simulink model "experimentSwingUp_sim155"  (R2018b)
settings: Solver=ode4  StartTime=0.0  StopTime=inf  FixedStep=1e-3  RelTol=1e-3
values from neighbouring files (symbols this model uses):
  K = lqr(sysd, Q_lqr, R_lqr)    [mainSkript_provedeniExperimentSwingUp.m]    (also in makeFBL.m = [0; -d_2*g*sin(th_1); -d_3*g*sin(th_2)]; mainSkript_simulaceLQG.m = lqr(sysd, Qk, Rk); mainSkript_LQGexperiment.m = lqr(sysd, Q, R); mainSkript_LQGexperiment_integral.m = lqr(sysd, Q, R))
  K1 = [K1(1 : idxL-rez_1); K1(idxL : idxH); K1(idxH+rez_2 : end)]    [mainSkript_provedeniExperimentSwingUp.m]    (also in mainSkript_provedeniSimulaceSwingUp.m = [K1(1 : idxL-rez); K1(idxL : idxH); K1(idxH+rez : end)])
  K2 = [K2(1 : idxL-rez_1); K2(idxL : idxH); K2(idxH+rez_2 : end)]    [mainSkript_provedeniExperimentSwingUp.m]    (also in mainSkript_provedeniSimulaceSwingUp.m = [K2(1 : idxL-rez); K2(idxL : idxH); K2(idxH+rez : end)])
  K3 = [K3(1 : idxL-rez_1); K3(idxL : idxH); K3(idxH+rez_2 : end)]    [mainSkript_provedeniExperimentSwingUp.m]    (also in mainSkript_provedeniSimulaceSwingUp.m = [K3(1 : idxL-rez); K3(idxL : idxH); K3(idxH+rez : end)])
  K4 = [K4(1 : idxL-rez_1); K4(idxL : idxH); K4(idxH+rez_2 : end)]    [mainSkript_provedeniExperimentSwingUp.m]    (also in mainSkript_provedeniSimulaceSwingUp.m = [K4(1 : idxL-rez); K4(idxL : idxH); K4(idxH+rez : end)])
  K5 = [K5(1 : idxL-rez_1); K5(idxL : idxH); K5(idxH+rez_2 : end)]    [mainSkript_provedeniExperimentSwingUp.m]    (also in mainSkript_provedeniSimulaceSwingUp.m = [K5(1 : idxL-rez); K5(idxL : idxH); K5(idxH+rez : end)])
  K6 = [K6(1 : idxL-rez_1); K6(idxL : idxH); K6(idxH+rez_2 : end)]    [mainSkript_provedeniExperimentSwingUp.m]    (also in mainSkript_provedeniSimulaceSwingUp.m = [K6(1 : idxL-rez); K6(idxL : idxH); K6(idxH+rez : end)])
  Ki = [Ki(1 : idxL-rez_1); Ki(idxL : idxH); Ki(idxH+rez_2 : end)]    [mainSkript_provedeniExperimentSwingUp.m]    (also in mainSkript_provedeniSimulaceSwingUp.m = [Ki(1 : idxL-rez); Ki(idxL : idxH); Ki(idxH+rez : end)])
  t_FB = [t_FB(1 : idxL-rez_1); t_FB(idxL : idxH); t_FB(idxH+rez_2 : end)]    [mainSkript_provedeniExperimentSwingUp.m]    (also in mainSkript_provedeniSimulaceSwingUp.m = [t_FB(1 : idxL-rez); t_FB(idxL : idxH); t_FB(idxH+rez : end))
  Ts = 1e-3    (= 0.001)    [mainSkript_provedeniExperimentSwingUp.m]    (also in mainSkript_rovniceSystemu.m; mainSkript_simulaceLQG.m; mainSkript_LQGexperiment.m; mainSkript_LQGexperiment_integral.m)
undefined symbols (not defined in the file or in its folder): DiscIntNeverNeededParam, Humusoft, MF624
libraries: sldrtlib x8, simulink x7, powerlib_meascontrol x3, sharedTrackingLibrary x2

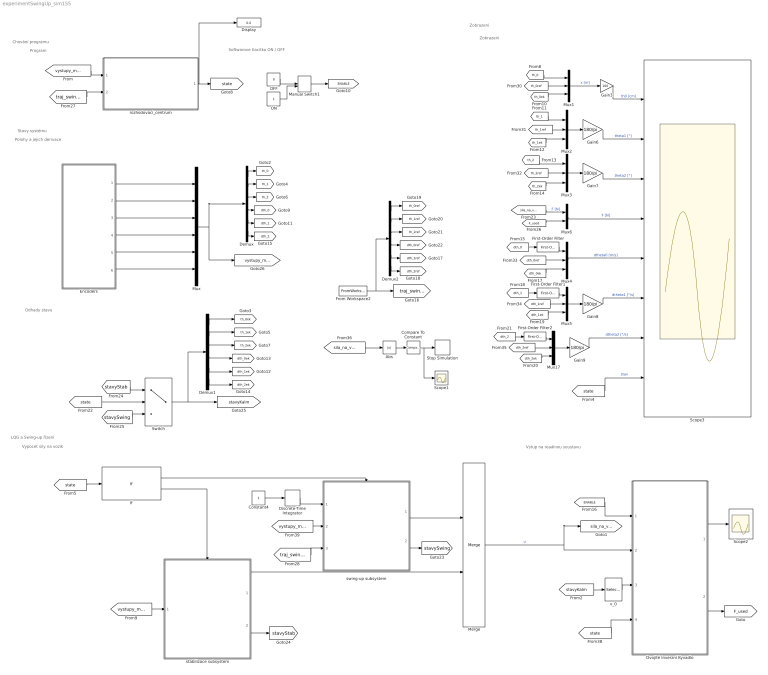
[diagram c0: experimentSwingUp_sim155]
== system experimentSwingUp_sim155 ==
  note: Odhady stavu
  note: Zobrazeni
  note: Chování programu
  note: LQG a Swing-up řízení
  note: Stavy systému
  note: Polohy a jejich derivace
  note: Softwarove tlacitko ON / OFF
  note: Program
  note: Vstup na reaálnou soustavu
  note: Vypocet sily na vozik
  note: Zobrazeni
  Abs : Abs
  Compare To Constant : simulink/Logic and Bit Operations/Compare To Constant  relop=>  const=35  OutDataTypeStr=boolean
  Constant4 : Constant
  Demux : Demux  Outputs=6
  Demux1 : Demux  Outputs=6
  Demux2 : Demux  Outputs=6
  Discrete-Time Integrator : DiscreteIntegrator  SampleTime=Ts  ICPrevOutput=DiscIntNeverNeededParam  ICPrevScaledInput=DiscIntNeverNeededParam
  Display : Display
  Dvojité Inverzní Kyvadlo : Subsystem
  Encoders : Subsystem
  First-Order Filter : powerlib_meascontrol/Filters/First-Order Filter  FilterType=Lowpass  Tc=4e-3  Ts=Ts  Initialize=on  Vac_Init=[0, 0, 60]  Vdc_Init=0  PlotResponse=off  FreqRange="[0,  200,  1]"
  First-Order Filter1 : powerlib_meascontrol/Filters/First-Order Filter  FilterType=Lowpass  Tc=6e-3  Ts=Ts  Initialize=on  Vac_Init=[0, 0, 60]  Vdc_Init=0  PlotResponse=off  FreqRange="[0,  200,  1]"
  First-Order Filter2 : powerlib_meascontrol/Filters/First-Order Filter  FilterType=Lowpass  Tc=6e-3  Ts=Ts  Initialize=on  Vac_Init=[0, 0, 60]  Vdc_Init=0  PlotResponse=off  FreqRange="[0,  200,  1]"
  From Workspace2 : FromWorkspace  VariableName=ref_traj  SampleTime=Ts
  Gain3 : Gain  Gain=100
  Gain{6..9} (4 alike) : Gain  Gain=180/pi
  If : If  IfExpression=u1 == 0  ElseIfExpressions=u1 == 1  ShowElse=off
  Manual Switch1 : ManualSwitch  CurrentSetting=0
  Merge : Merge
  Mux : Mux  Inputs=6
  Mux{1..5,17} (6 alike) : Mux  Inputs=3
  Mux6 : Mux  Inputs=2
  OFF : Constant  Value=0
  ON : Constant
  Scope1 : Scope
  Scope2 : Scope
  Scope3 : Scope  NumInputPorts=8
  Stop Simulation : Stop
  Switch : Switch  Criteria=u2 > Threshold
  rozhodovaci_centrum : Subsystem
  stabilizace subsystem : Subsystem  TreatAsAtomicUnit=on
  swing-up subsystem : Subsystem  TreatAsAtomicUnit=on
  v_0 : Selector  InputPortWidth=6  IndexOptions=Index vector (dialog)  Indices=[4]  OutputSizes=1
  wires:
  OFF/1 -> Manual Switch1/1
  ON/1 -> Manual Switch1/2
  Manual Switch1/1 -> [ENABLE]
  [ENABLE] -> Dvojité Inverzní Kyvadlo/1(ENABLE)
  Dvojité Inverzní Kyvadlo/1(sat_flag) -> Scope2/1
  Dvojité Inverzní Kyvadlo/2(F_used [N]) -> [F_used]
  If/2 -> stabilizace subsystem/Action
  Discrete-Time Integrator/1 -> swing-up subsystem/1(cas Swing-upu [s])
  If/1 -> swing-up subsystem/Action
  stabilizace subsystem/1(sila na vozik [N]) -> Merge/2
  [stavyKalm] -> v_0/1
  [vystupy_mereni] -> rozhodovaci_centrum/1(stavySystemu)
  [state] -> Scope3/8  "stav"
  Mux/1 -> [vystupy_mereni], Demux/1
  Switch/1 -> Demux1/1, [stavyKalm]
  Demux/1 -> [th_0]
  Demux1/1 -> [th_0ek]
  Demux/2 -> [th_1]
  Demux1/2 -> [th_1ek]
  Demux/3 -> [th_2]
  Demux1/3 -> [th_2ek]
  Demux/4 -> [dth_0]
  Demux/5 -> [dth_1]
  Demux1/5 -> [dth_1ek]
  Demux1/4 -> [dth_0ek]
  Demux1/6 -> [dth_2ek]
  Demux/6 -> [dth_2]
  Constant4/1 -> Discrete-Time Integrator/1
  Compare To Constant/1 -> Scope1/1, Stop Simulation/1
  Encoders/1(th0 [m]) -> Mux/1
  Encoders/2(th1 [rad]) -> Mux/2
  Encoders/3(th2 [rad]) -> Mux/3
  Encoders/5(dth1 [rad/s]) -> Mux/5
  Encoders/6(dth2 [rad/s]) -> Mux/6
  Mux17/1 -> Gain9/1
  Gain8/1 -> Scope3/6  "dtheta1 [°/s]"
  [th_2] -> Mux3/1
  [dth_0] -> First-Order Filter/1
  [dth_0ref] -> Mux4/2
  [th_0ref] -> Mux1/2
  [dth_1ref] -> Mux5/2
  Gain7/1 -> Scope3/3  "theta2 [°]"
  Gain6/1 -> Scope3/2  "theta1 [°]"
  Mux5/1 -> Gain8/1
  [th_2ek] -> Mux3/3
  Mux4/1 -> Scope3/5  "dtheta0 [m/s]"
  [th_0] -> Mux1/1
  [th_2ref] -> Mux3/2
  Gain9/1 -> Scope3/7  "dtheta2 [°/s]"
  Mux1/1 -> Gain3/1  "x [m]"
  [dth_2ek] -> Mux17/3
  [dth_1ek] -> Mux5/3
  Mux2/1 -> Gain6/1
  [dth_0ek] -> Mux4/3
  [dth_2ref] -> Mux17/2
  [th_1ref] -> Mux2/2
  [th_1ek] -> Mux2/3
  Mux3/1 -> Gain7/1
  [th_1] -> Mux2/1
  [th_0ek] -> Mux1/3
  Gain3/1 -> Scope3/1  "th0 [cm]"
  [sila_na_vozik] -> Mux6/1  "F [N]"
  Mux6/1 -> Scope3/4  "F [N]"
  [F_used] -> Mux6/2
  [traj_swingUp] -> rozhodovaci_centrum/2(trajektorieSwingUp)
  [traj_swingUp] -> swing-up subsystem/3(trajektorie swing-up)
  Demux2/6 -> [dth_2ref]
  Demux2/5 -> [dth_1ref]
  Demux2/4 -> [dth_0ref]
  Demux2/3 -> [th_2ref]
  Demux2/2 -> [th_1ref]
  Demux2/1 -> [th_0ref]
  From Workspace2/1 -> Demux2/1, [traj_swingUp]
  [state] -> If/1
  Abs/1 -> Compare To Constant/1
  [sila_na_vozik] -> Abs/1
  swing-up subsystem/1(sila na vozik [N]) -> Merge/1
  rozhodovaci_centrum/1(error_state) -> [state], Display/1
  Encoders/4(dth0 [m/s]) -> Mux/4
  First-Order Filter/1 -> Mux4/1
  [dth_1] -> First-Order Filter1/1
  First-Order Filter1/1 -> Mux5/1
  [dth_2] -> First-Order Filter2/1
  First-Order Filter2/1 -> Mux17/1
  [state] -> Dvojité Inverzní Kyvadlo/4(stav)
  [vystupy_mereni] -> swing-up subsystem/2(mereni)
  swing-up subsystem/2(stavyKalm) -> [stavySwing]
  [vystupy_mereni] -> stabilizace subsystem/1(mereni)
  stabilizace subsystem/2(stavy) -> [stavyStab]
  [stavyStab] -> Switch/1
  [state] -> Switch/2
  [stavySwing] -> Switch/3
  v_0/1 -> Dvojité Inverzní Kyvadlo/3(v [m/s])
  Merge/1 -> [sila_na_vozik], Dvojité Inverzní Kyvadlo/2(F_in [N])  "u"

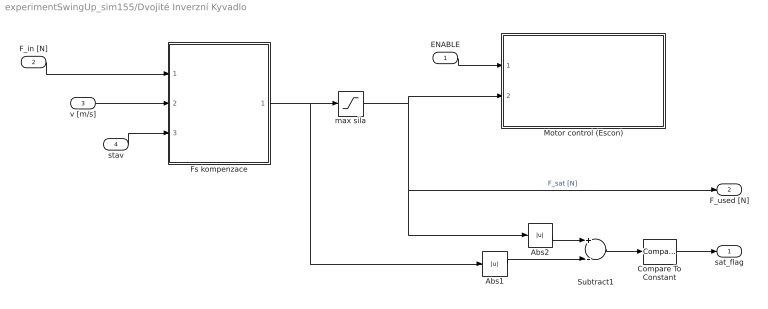
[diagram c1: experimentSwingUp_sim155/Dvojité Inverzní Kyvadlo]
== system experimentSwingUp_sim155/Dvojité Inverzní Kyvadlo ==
  ENABLE : Inport
  F_in [N] : Inport  Port=2
  v [m/s] : Inport  Port=3
  stav : Inport  Port=4
  Abs1 : Abs
  Abs2 : Abs
  Compare To Constant : simulink/Logic and Bit Operations/Compare To Constant  relop=>  const=1e-8  OutDataTypeStr=boolean
  Fs kompenzace : Subsystem
  Motor control (Escon) : Subsystem
  Subtract1 : Sum  Inputs=+-
  max sila : Saturate  UpperLimit=50  LowerLimit=-50
  sat_flag : Outport
  F_used [N] : Outport  Port=2
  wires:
  ENABLE/1 -> Motor control (Escon)/1(ENABLE)
  v [m/s]/1 -> Fs kompenzace/2(v [m/s])
  F_in [N]/1 -> Fs kompenzace/1(F_in [N])
  Compare To Constant/1 -> sat_flag/1
  Subtract1/1 -> Compare To Constant/1
  Abs1/1 -> Subtract1/2
  max sila/1 -> Motor control (Escon)/2(Ref strength [N]), F_used [N]/1, Abs2/1  "F_sat [N]"
  Abs2/1 -> Subtract1/1
  Fs kompenzace/1(F_out [N]) -> Abs1/1, max sila/1
  stav/1 -> Fs kompenzace/3(stav)

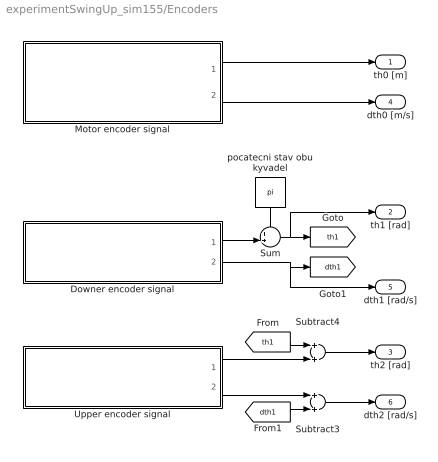
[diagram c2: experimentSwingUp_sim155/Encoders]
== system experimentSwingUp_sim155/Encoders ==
  Downer encoder signal : Subsystem
  Motor encoder signal : Subsystem
  Subtract3 : Sum
  Subtract4 : Sum
  Sum : Sum  Inputs=++|
  Upper encoder signal : Subsystem
  pocatecni stav obu kyvadel : Constant  Value=pi
  th0 [m] : Outport
  th1 [rad] : Outport  Port=2
  th2 [rad] : Outport  Port=3
  dth0 [m/s] : Outport  Port=4
  dth1 [rad/s] : Outport  Port=5
  dth2 [rad/s] : Outport  Port=6
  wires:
  pocatecni stav obu kyvadel/1 -> Sum/1
  Downer encoder signal/1(phi [rad]) -> Sum/2
  Sum/1 -> th1 [rad]/1, [th1]
  Downer encoder signal/2(omega [rad/s]) -> dth1 [rad/s]/1, [dth1]
  Upper encoder signal/1(phi [rad]) -> Subtract4/2
  Upper encoder signal/2(omega [rad/s]) -> Subtract3/1
  [th1] -> Subtract4/1
  [dth1] -> Subtract3/2
  Subtract4/1 -> th2 [rad]/1
  Subtract3/1 -> dth2 [rad/s]/1
  Motor encoder signal/1(x [m]) -> th0 [m]/1
  Motor encoder signal/2(v [m/s]) -> dth0 [m/s]/1

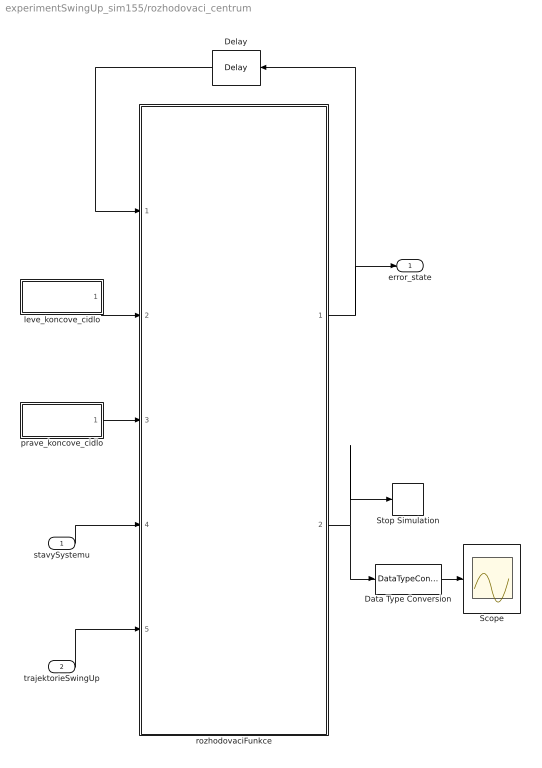
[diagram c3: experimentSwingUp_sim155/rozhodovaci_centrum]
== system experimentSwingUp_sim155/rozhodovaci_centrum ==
  stavySystemu : Inport
  trajektorieSwingUp : Inport  Port=2
  Data Type Conversion : DataTypeConversion  OutDataTypeStr=double
  Delay : Delay  DelayLength=1  InitialCondition=0  UseCircularBuffer=on  SampleTime=Ts
  Scope : Scope
  Stop Simulation : Stop
  leve_koncove_cidlo : Subsystem
  prave_koncove_cidlo : Subsystem
  rozhodovaciFunkce : MATLAB Function  TreatAsAtomicUnit=on
  error_state : Outport
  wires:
  rozhodovaciFunkce/1(state) -> Delay/1, error_state/1
  rozhodovaciFunkce/2(error) -> Stop Simulation/1, Data Type Conversion/1
  Delay/1 -> rozhodovaciFunkce/1(last_state)
  Data Type Conversion/1 -> Scope/1
  leve_koncove_cidlo/1(NOK) -> rozhodovaciFunkce/2(leftSens)
  prave_koncove_cidlo/1(NOK) -> rozhodovaciFunkce/3(rightSens)
  stavySystemu/1 -> rozhodovaciFunkce/4(stavySystemu)
  trajektorieSwingUp/1 -> rozhodovaciFunkce/5(traj)

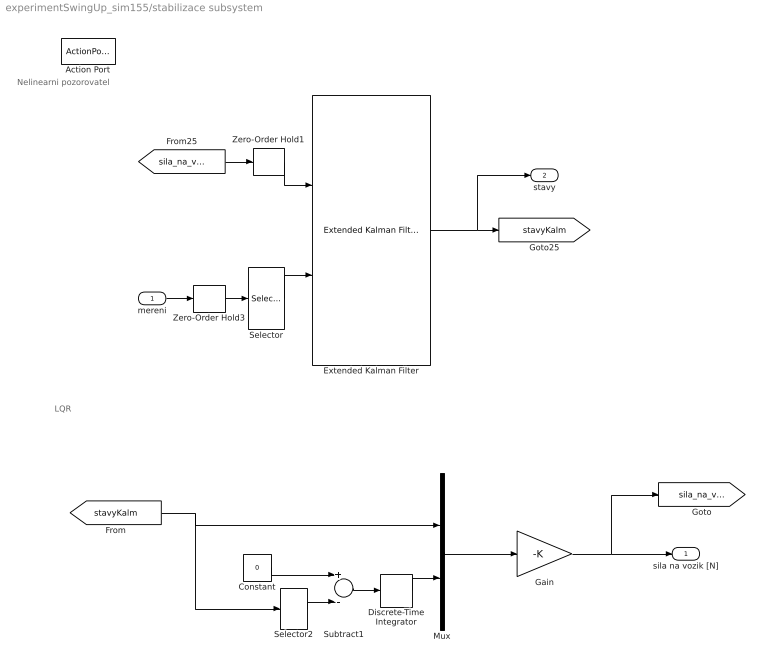
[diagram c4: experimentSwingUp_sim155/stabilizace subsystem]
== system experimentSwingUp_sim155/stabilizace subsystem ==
  note: LQR
  note: Nelinearni pozorovatel
  mereni : Inport
  Action Port : ActionPort  ActionType=elseif
  Constant : Constant  Value=0
  Discrete-Time Integrator : DiscreteIntegrator  SampleTime=Ts  ICPrevOutput=DiscIntNeverNeededParam  ICPrevScaledInput=DiscIntNeverNeededParam
  Extended Kalman Filter : sharedTrackingLibrary/Extended Kalman Filter  StateTransitionFcn=nonLinKalmFcn_pn0  HasStateTransitionJacobianFcn=on  StateTransitionJacobianFcn=countJacobDIP_pn0  HasAdditiveProcessNoise=Additive  ProcessNoise=Q_stab  HasTimeVaryingProcessNoise=off  HasStateTransitionFcnExtraArgument=1  InitialState=q_0  InitialStateCovariance=1e-6*eye(6)  MeasurementFcn1=mereniStavuKalm  HasMeasurementJacobianFcn1=off  HasMeasurementEnablePort1=off  HasAdditiveMeasurementNoise1=Additive  MeasurementNoise1=R_stab  HasTimeVaryingMeasurementNoise1=off  HasMeasurementFcnExtraArgument1=0  MeasurementFcn2=myMeasurementFcn  HasMeasurementJacobianFcn2=off  HasMeasurementEnablePort2=off  HasAdditiveMeasurementNoise2=Additive  MeasurementNoise2=1  HasTimeVaryingMeasurementNoise2=off  HasMeasurementFcnExtraArgument2=0  MeasurementFcn3=myMeasurementFcn  HasMeasurementJacobianFcn3=off  HasMeasurementEnablePort3=off  HasAdditiveMeasurementNoise3=Additive  MeasurementNoise3=1  HasTimeVaryingMeasurementNoise3=off  HasMeasurementFcnExtraArgument3=0  MeasurementFcn4=myMeasurementFcn  HasMeasurementJacobianFcn4=off  HasMeasurementEnablePort4=off  HasAdditiveMeasurementNoise4=Additive  MeasurementNoise4=1  HasTimeVaryingMeasurementNoise4=off  HasMeasurementFcnExtraArgument4=0  MeasurementFcn5=myMeasurementFcn  HasMeasurementJacobianFcn5=off  HasMeasurementEnablePort5=off  HasAdditiveMeasurementNoise5=Additive  MeasurementNoise5=1  HasTimeVaryingMeasurementNoise5=off  HasMeasurementFcnExtraArgument5=0  EnableMultirate=off  StateTransitionFcnSampleTime=1  MeasurementFcn1SampleTime=1  MeasurementFcn2SampleTime=1  MeasurementFcn3SampleTime=1  MeasurementFcn4SampleTime=1  MeasurementFcn5SampleTime=1  UseCurrentEstimator=on  OutputStateCovariance=off  DataType=double  SampleTime=Ts  NumberOfMeasurements=1
  Gain : Gain  Gain=-K  Multiplication=Matrix(K*u) (u vector)
  Mux : Mux  Inputs=2
  Selector : Selector  InputPortWidth=6  IndexOptions=Index vector (dialog)  Indices=[1:3]  OutputSizes=1
  Selector2 : Selector  InputPortWidth=6  IndexOptions=Index vector (dialog)  Indices=[1]  OutputSizes=1
  Subtract1 : Sum  Inputs=+-
  Zero-Order Hold1 : ZeroOrderHold  SampleTime=Ts
  Zero-Order Hold3 : ZeroOrderHold  SampleTime=Ts
  sila na vozik [N] : Outport
  stavy : Outport  Port=2
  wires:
  Selector2/1 -> Subtract1/2
  Subtract1/1 -> Discrete-Time Integrator/1
  Mux/1 -> Gain/1
  Discrete-Time Integrator/1 -> Mux/2
  Constant/1 -> Subtract1/1
  Gain/1 -> [sila_na_vozik], sila na vozik [N]/1
  Zero-Order Hold3/1 -> Selector/1
  [sila_na_vozik] -> Zero-Order Hold1/1
  Selector/1 -> Extended Kalman Filter/2
  mereni/1 -> Zero-Order Hold3/1
  Extended Kalman Filter/1 -> stavy/1, [stavyKalm]
  Zero-Order Hold1/1 -> Extended Kalman Filter/1
  [stavyKalm] -> Selector2/1, Mux/1

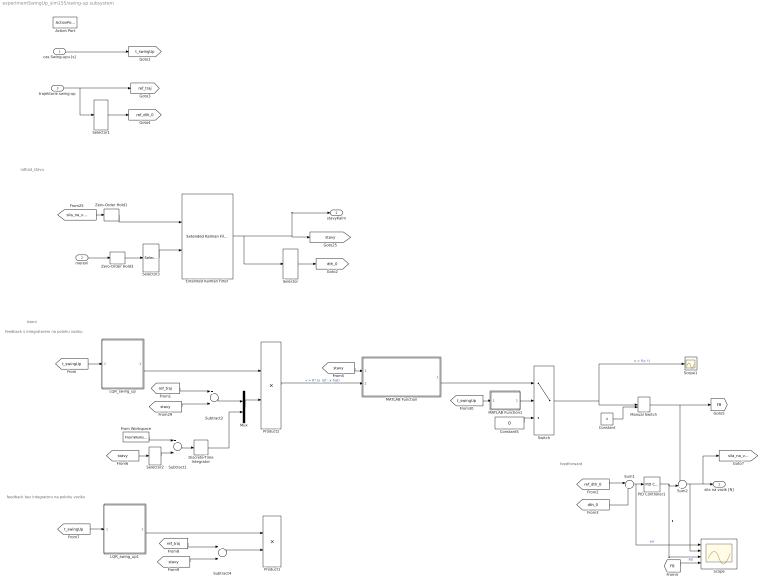
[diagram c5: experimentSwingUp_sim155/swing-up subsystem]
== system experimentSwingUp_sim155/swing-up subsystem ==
  note: odhad_stavu
  note: rizeni
  note: feedback s integratorem na polohu voziku
  note: feedforward
  note: feedback bez integratoru na polohu voziku
  cas Swing-upu [s] : Inport
  mereni : Inport  Port=2
  trajektorie swing-up : Inport  Port=3
  Action Port : ActionPort  ActionType=then
  Constant : Constant  Value=0
  Constant5 : Constant  Value=0
  Discrete-Time Integrator : DiscreteIntegrator  SampleTime=Ts  ICPrevOutput=DiscIntNeverNeededParam  ICPrevScaledInput=DiscIntNeverNeededParam
  Extended Kalman Filter : sharedTrackingLibrary/Extended Kalman Filter  StateTransitionFcn=nonLinKalmFcn_pn155  HasStateTransitionJacobianFcn=on  StateTransitionJacobianFcn=countJacobDIP_pn155  HasAdditiveProcessNoise=Additive  ProcessNoise=Q_swing  HasTimeVaryingProcessNoise=off  HasStateTransitionFcnExtraArgument=1  InitialState=q_0  InitialStateCovariance=1e-6*eye(6)  MeasurementFcn1=mereniStavuKalm  HasMeasurementJacobianFcn1=off  HasMeasurementEnablePort1=off  HasAdditiveMeasurementNoise1=Additive  MeasurementNoise1=R_swing  HasTimeVaryingMeasurementNoise1=off  HasMeasurementFcnExtraArgument1=0  MeasurementFcn2=myMeasurementFcn  HasMeasurementJacobianFcn2=off  HasMeasurementEnablePort2=off  HasAdditiveMeasurementNoise2=Additive  MeasurementNoise2=1  HasTimeVaryingMeasurementNoise2=off  HasMeasurementFcnExtraArgument2=0  MeasurementFcn3=myMeasurementFcn  HasMeasurementJacobianFcn3=off  HasMeasurementEnablePort3=off  HasAdditiveMeasurementNoise3=Additive  MeasurementNoise3=1  HasTimeVaryingMeasurementNoise3=off  HasMeasurementFcnExtraArgument3=0  MeasurementFcn4=myMeasurementFcn  HasMeasurementJacobianFcn4=off  HasMeasurementEnablePort4=off  HasAdditiveMeasurementNoise4=Additive  MeasurementNoise4=1  HasTimeVaryingMeasurementNoise4=off  HasMeasurementFcnExtraArgument4=0  MeasurementFcn5=myMeasurementFcn  HasMeasurementJacobianFcn5=off  HasMeasurementEnablePort5=off  HasAdditiveMeasurementNoise5=Additive  MeasurementNoise5=1  HasTimeVaryingMeasurementNoise5=off  HasMeasurementFcnExtraArgument5=0  EnableMultirate=off  StateTransitionFcnSampleTime=1  MeasurementFcn1SampleTime=1  MeasurementFcn2SampleTime=1  MeasurementFcn3SampleTime=1  MeasurementFcn4SampleTime=1  MeasurementFcn5SampleTime=1  UseCurrentEstimator=on  OutputStateCovariance=off  DataType=double  SampleTime=Ts  NumberOfMeasurements=1
  From Workspace : FromWorkspace  VariableName=theta0_str  SampleTime=Ts
  LQR_swing_up : Subsystem
  LQR_swing_up1 : Subsystem  Commented=on
  MATLAB Function : MATLAB Function  TreatAsAtomicUnit=on
  MATLAB Function1 : MATLAB Function  TreatAsAtomicUnit=on
  Manual Switch : ManualSwitch
  Mux : Mux  Inputs=2
  PID Controller1 : simulink/Continuous/PID Controller  Controller=PID  Form=Parallel  TimeDomain=Discrete-time  SampleTime=Ts  IntegratorMethod=Forward Euler  FilterMethod=Forward Euler  ControllerParametersSource=internal  P=520  I=1610  D=0  UseFilter=on  N=100  TunerSelectOption=Transfer Function Based (PID Tuner App)  InitialConditionSource=internal  InitialConditionForIntegrator=0  InitialConditionForFilter=0  DifferentiatorICPrevScaledInput=0  ExternalReset=none  TrackingMode=off  Kt=1  LimitOutput=off  UpperSaturationLimit=inf  LowerSaturationLimit=-inf  LinearizeAsGain=on  AntiWindupMode=none  Kb=1  POutMin=[]  POutMax=[]  IOutMin=[]  IOutMax=[]  DOutMin=[]  DOutMax=[]  NOutMin=[]  NOutMax=[]  SumOutMin=[]  SumOutMax=[]  SaturationOutMin=[]  SaturationOutMax=[]  PParamMin=[]  PParamMax=[]  IParamMin=[]  IParamMax=[]  DParamMin=[]  DParamMax=[]  NParamMin=[]  NParamMax=[]  KbParamMin=[]  KbParamMax=[]  KtParamMin=[]  KtParamMax=[]  KbOutMin=[]  KbOutMax=[]  KtOutMin=[]  KtOutMax=[]  IntegratorOutMin=[]  IntegratorOutMax=[]  FilterOutMin=[]  FilterOutMax=[]  SumI1OutMin=[]  SumI1OutMax=[]  SumI2OutMin=[]  SumI2OutMax=[]  SumI3OutMin=[]  SumI3OutMax=[]  SumI4OutMin=[]  SumI4OutMax=[]  SumDOutMin=[]  SumDOutMax=[]  DifferentiatorOutMin=[]  DifferentiatorOutMax=[]  FilterDiffOutCoefMin=[]  FilterDiffOutCoefMax=[]  ReciprocalOutMin=[]  ReciprocalOutMax=[]  SumDenOutMin=[]  SumDenOutMax=[]  SumNumOutMin=[]  SumNumOutMax=[]  DivideOutMin=[]  DivideOutMax=[]  IntegratorContinuousStateAttributes=''  IntegratorStateMustResolveToSignalObject=off  IntegratorRTWStateStorageClass=Auto  FilterContinuousStateAttributes=''  FilterStateMustResolveToSignalObject=off  FilterRTWStateStorageClass=Auto  ParallelPVariant=InternalParameters  IdealPVariant=Disabled  IVariant=InternalParameters  DVariant=InternalParameters  IntegratorVariant=Discrete  SatVariant=Disabled  AWVariant=Passthrough  PCopyVariant=Disabled  TRVariant=Disabled  FdbkBlocksVariant=Forward  IdealPFdbkVariant=Disabled  SatFdbkVariant=Disabled  DerivativeFilterVariant=ForwardEulerFilter  NVariant=InternalParameters  NCopyVariant=Disabled  FilterICVariant=InternalICsFilter  IntegratorICVariant=InternalICs  ExternalResetVariant=Disabled  TRSumVariant=Passthrough  SumFdbkVariant=Disabled  SumVariant=Sum_PID
  Product1 : Product  Commented=on  Multiplication=Matrix(*)
  Product2 : Product  Multiplication=Matrix(*)
  Scope : Scope  NumInputPorts=4
  Scope1 : Scope
  Selector : Selector  InputPortWidth=6  IndexOptions=Index vector (dialog)  Indices=[4]  OutputSizes=1
  Selector1 : Selector  InputPortWidth=6  IndexOptions=Index vector (dialog)  Indices=[4]  OutputSizes=1
  Selector2 : Selector  InputPortWidth=6  IndexOptions=Index vector (dialog)  Indices=[1]  OutputSizes=1
  Selector3 : Selector  InputPortWidth=6  IndexOptions=Index vector (dialog)  Indices=[1:3]  OutputSizes=1
  Subtract1 : Sum  Inputs=+-
  Subtract2 : Sum  Inputs=+-
  Subtract4 : Sum  Commented=on  Inputs=+-
  Sum1 : Sum  Inputs=|+-
  Sum2 : Sum  Inputs=++|
  Switch : Switch  Criteria=u2 ~= 0
  Zero-Order Hold1 : ZeroOrderHold  SampleTime=Ts
  Zero-Order Hold3 : ZeroOrderHold  SampleTime=Ts
  sila na vozik [N] : Outport
  stavyKalm : Outport  Port=2
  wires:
  Sum2/1 -> Scope/2, [sila_na_vozik], sila na vozik [N]/1
  Sum1/1 -> Scope/1, PID Controller1/1  "err"
  [ref_dth_0] -> Sum1/1
  PID Controller1/1 -> Scope/3, Sum2/2  "FF"
  [stavy] -> Subtract2/2
  Constant5/1 -> Switch/3
  [t_swingUp] -> MATLAB Function1/1(time)
  [dth_0] -> Sum1/2
  cas Swing-upu [s]/1 -> [t_swingUp]
  [t_swingUp] -> LQR_swing_up/1(t)
  Selector/1 -> [dth_0]
  trajektorie swing-up/1 -> Selector1/1, [ref_traj]
  Selector1/1 -> [ref_dth_0]
  [ref_traj] -> Subtract2/1
  LQR_swing_up/1(K(t)) -> Product2/1
  MATLAB Function1/1(on) -> Switch/2
  Switch/1 -> Scope1/1, Manual Switch/1  "u = f(x, t)"
  Constant/1 -> Manual Switch/2
  Manual Switch/1 -> [FB], Sum2/1
  [FB] -> Scope/4  "FB"
  MATLAB Function/1(u) -> Switch/1
  [stavy] -> MATLAB Function/1(y)
  Mux/1 -> Product2/2
  Subtract2/1 -> Mux/1
  From Workspace/1 -> Subtract1/1
  Selector2/1 -> Subtract1/2
  [stavy] -> Selector2/1
  Subtract1/1 -> Discrete-Time Integrator/1
  Discrete-Time Integrator/1 -> Mux/2
  mereni/1 -> Zero-Order Hold3/1
  Zero-Order Hold3/1 -> Selector3/1
  Selector3/1 -> Extended Kalman Filter/2
  Extended Kalman Filter/1 -> Selector/1, stavyKalm/1, [stavy]
  Zero-Order Hold1/1 -> Extended Kalman Filter/1
  [sila_na_vozik] -> Zero-Order Hold1/1
  [stavy] -> Subtract4/2
  LQR_swing_up1/1(K(t)) -> Product1/1
  [t_swingUp] -> LQR_swing_up1/1(t)
  [ref_traj] -> Subtract4/1
  Subtract4/1 -> Product1/2
  Product2/1 -> MATLAB Function/2(v)  "v = K* (x_ref - x_hat)"

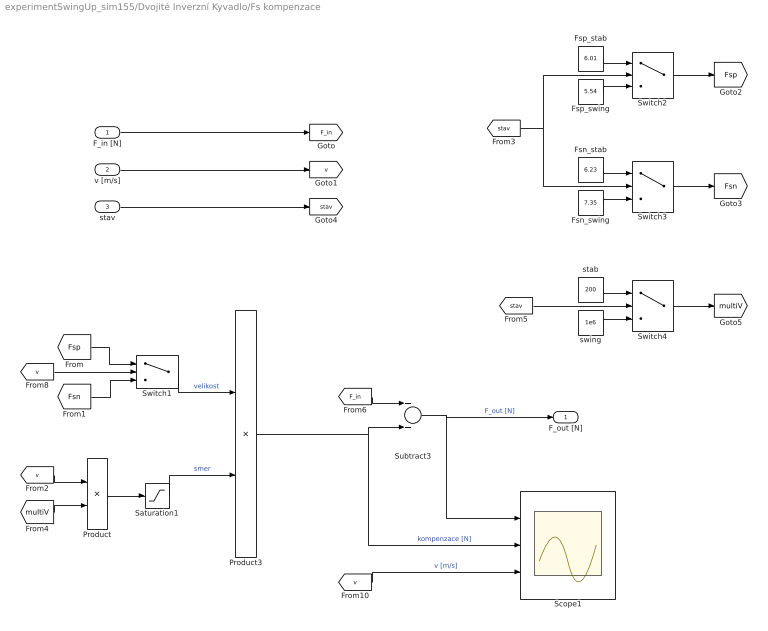
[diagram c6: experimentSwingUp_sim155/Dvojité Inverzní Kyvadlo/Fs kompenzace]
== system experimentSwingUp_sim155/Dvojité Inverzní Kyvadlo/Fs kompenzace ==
  F_in [N] : Inport
  v [m/s] : Inport  Port=2
  stav : Inport  Port=3
  Fsn_stab : Constant  Value=6.23
  Fsn_swing : Constant  Value=7.35
  Fsp_stab : Constant  Value=6.01
  Fsp_swing : Constant  Value=5.54
  Product : Product
  Product3 : Product
  Saturation1 : Saturate  UpperLimit=1  LowerLimit=-1
  Scope1 : Scope  NumInputPorts=3
  Subtract3 : Sum
  Switch1 : Switch
  Switch2 : Switch  Criteria=u2 > Threshold
  Switch3 : Switch  Criteria=u2 > Threshold
  Switch4 : Switch  Criteria=u2 > Threshold
  stab : Constant  Value=200
  swing : Constant  Value=1e6
  F_out [N] : Outport
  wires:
  F_in [N]/1 -> [F_in]
  v [m/s]/1 -> [v]
  [Fsn] -> Switch1/3
  [v] -> Switch1/2
  [Fsp] -> Switch1/1
  [F_in] -> Subtract3/1
  [v] -> Scope1/3  "v [m/s]"
  Subtract3/1 -> F_out [N]/1, Scope1/1  "F_out [N]"
  Saturation1/1 -> Product3/2  "smer"
  Product3/1 -> Subtract3/2, Scope1/2  "kompenzace [N]"
  Product/1 -> Saturation1/1
  Switch1/1 -> Product3/1  "velikost"
  [stav] -> Switch3/2, Switch2/2
  Fsp_swing/1 -> Switch2/3
  Fsn_swing/1 -> Switch3/3
  Switch2/1 -> [Fsp]
  Switch3/1 -> [Fsn]
  Fsp_stab/1 -> Switch2/1
  Fsn_stab/1 -> Switch3/1
  stav/1 -> [stav]
  [v] -> Product/1
  [multiV] -> Product/2
  [stav] -> Switch4/2
  swing/1 -> Switch4/3
  stab/1 -> Switch4/1
  Switch4/1 -> [multiV]

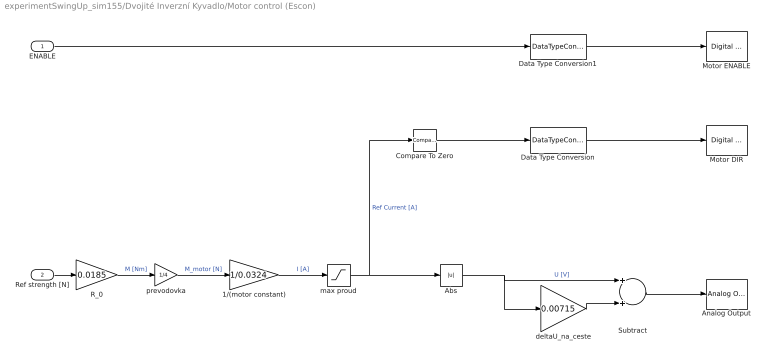
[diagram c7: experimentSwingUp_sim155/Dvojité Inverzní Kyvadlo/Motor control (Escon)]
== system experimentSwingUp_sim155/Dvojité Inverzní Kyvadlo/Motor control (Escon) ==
  ENABLE : Inport
  Ref strength [N] : Inport  Port=2
  1/(motor constant) : Gain  Gain=1/0.0324
  Abs : Abs
  Analog Output : sldrtlib/Analog Output  SampleTime=Ts  MaxMissedTicks=1e6  ShowMissedTicks=off  YieldWhenWaiting=off  DrvName=Humusoft/MF624  DrvAddress=4294967295  DrvOptions=0  Channels=6  RangeMode=1  VoltRange=1  InitialValue=0  FinalValue=0
  Compare To Zero : simulink/Logic and Bit Operations/Compare To Zero  relop=>=  OutDataTypeStr=boolean
  Data Type Conversion : DataTypeConversion  OutDataTypeStr=boolean
  Data Type Conversion1 : DataTypeConversion  OutDataTypeStr=boolean
  Motor DIR : sldrtlib/Digital Output  SampleTime=Ts  MaxMissedTicks=1e6  ShowMissedTicks=off  YieldWhenWaiting=off  DrvName=Humusoft/MF624  DrvAddress=4294967295  DrvOptions=0  Channels=5  BitMode=1  InitialValue=0  FinalValue=0
  Motor ENABLE : sldrtlib/Digital Output  SampleTime=Ts  MaxMissedTicks=1e6  ShowMissedTicks=off  YieldWhenWaiting=off  DrvName=Humusoft/MF624  DrvAddress=4294967295  DrvOptions=0  Channels=2  BitMode=1  InitialValue=0  FinalValue=0
  R_0 : Gain  Gain=0.0185
  Subtract : Sum
  deltaU_na_ceste : Gain  Gain=0.00715
  max proud : Saturate  UpperLimit=10  LowerLimit=-10
  prevodovka : Gain  Gain=1/4
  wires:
  Compare To Zero/1 -> Data Type Conversion/1
  Data Type Conversion1/1 -> Motor ENABLE/1
  1/(motor constant)/1 -> max proud/1  "I [A]"
  max proud/1 -> Abs/1, Compare To Zero/1  "Ref Current [A]"
  Ref strength [N]/1 -> R_0/1
  ENABLE/1 -> Data Type Conversion1/1
  R_0/1 -> prevodovka/1  "M [Nm]"
  prevodovka/1 -> 1/(motor constant)/1  "M_motor [N]"
  Data Type Conversion/1 -> Motor DIR/1
  Subtract/1 -> Analog Output/1
  deltaU_na_ceste/1 -> Subtract/2
  Abs/1 -> Subtract/1, deltaU_na_ceste/1  "U [V]"

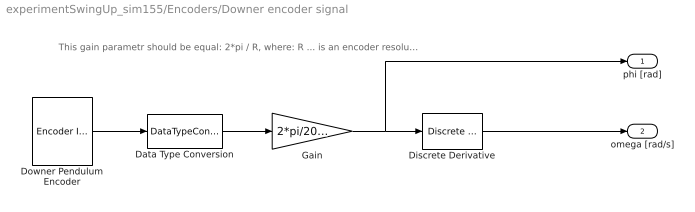
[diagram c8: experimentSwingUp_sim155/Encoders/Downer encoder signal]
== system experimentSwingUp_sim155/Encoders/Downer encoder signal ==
  note: This gain parametr should be equal: 2*pi / R, where: R ... is an encoder resolution
  Data Type Conversion : DataTypeConversion  OutDataTypeStr=double
  Discrete Derivative : simulink/Discrete/Discrete Derivative  gainval=1.0  ICPrevScaledInput=0.0  OutMin=[]  OutMax=[]  OutDataType=fixdt(1, 16)  OutScaling=2^-10  DoSatur=off
  Downer Pendulum Encoder : sldrtlib/Encoder Input  SampleTime=Ts  MaxMissedTicks=1e8  ShowMissedTicks=off  YieldWhenWaiting=off  DrvName=Humusoft/MF624  DrvAddress=4294967295  DrvOptions=0  Channels=2  QuadMode=3  IndexPulse=1  InputFilter=Inf  DataType=7
  Gain : Gain  Gain=2*pi/2048
  phi [rad] : Outport
  omega [rad/s] : Outport  Port=2
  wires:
  Downer Pendulum Encoder/1 -> Data Type Conversion/1
  Discrete Derivative/1 -> omega [rad/s]/1
  Data Type Conversion/1 -> Gain/1
  Gain/1 -> Discrete Derivative/1, phi [rad]/1

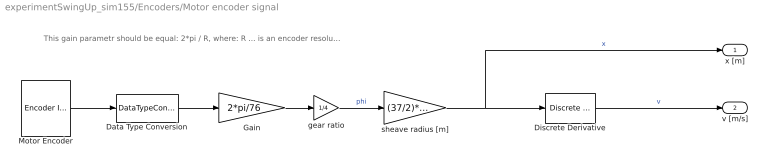
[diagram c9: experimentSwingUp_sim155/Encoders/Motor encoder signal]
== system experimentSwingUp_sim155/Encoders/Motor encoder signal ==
  note: This gain parametr should be equal: 2*pi / R, where: R ... is an encoder resolution
  Data Type Conversion : DataTypeConversion  OutDataTypeStr=double
  Discrete Derivative : simulink/Discrete/Discrete Derivative  gainval=1.0  ICPrevScaledInput=0.0  OutMin=[]  OutMax=[]  OutDataType=fixdt(1, 16)  OutScaling=2^-10  DoSatur=off
  Gain : Gain  Gain=2*pi/76
  Motor Encoder : sldrtlib/Encoder Input  SampleTime=Ts  MaxMissedTicks=1e8  ShowMissedTicks=off  YieldWhenWaiting=off  DrvName=Humusoft/MF624  DrvAddress=4294967295  DrvOptions=0  Channels=3  QuadMode=3  IndexPulse=1  InputFilter=Inf  DataType=7
  gear ratio : Gain  Gain=1/4
  sheave radius [m] : Gain  Gain=(37/2)*1e-3
  x [m] : Outport
  v [m/s] : Outport  Port=2
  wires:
  Motor Encoder/1 -> Data Type Conversion/1
  Discrete Derivative/1 -> v [m/s]/1  "v"
  Data Type Conversion/1 -> Gain/1
  Gain/1 -> gear ratio/1
  sheave radius [m]/1 -> Discrete Derivative/1, x [m]/1  "x"
  gear ratio/1 -> sheave radius [m]/1  "phi"

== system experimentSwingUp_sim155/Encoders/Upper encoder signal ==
  note: This gain parametr should be equal: 2*pi / R, where: R ... is an encoder resolution
  Data Type Conversion : DataTypeConversion  OutDataTypeStr=double
  Discrete Derivative : simulink/Discrete/Discrete Derivative  gainval=1.0  ICPrevScaledInput=0.0  OutMin=[]  OutMax=[]  OutDataType=fixdt(1, 16)  OutScaling=2^-10  DoSatur=off
  Gain : Gain  Gain=2*pi/2048
  Upper Pendulum Encoder : sldrtlib/Encoder Input  SampleTime=Ts  MaxMissedTicks=1e8  ShowMissedTicks=off  YieldWhenWaiting=off  DrvName=Humusoft/MF624  DrvAddress=4294967295  DrvOptions=0  Channels=4  QuadMode=3  IndexPulse=1  InputFilter=Inf  DataType=7
  phi [rad] : Outport
  omega [rad/s] : Outport  Port=2
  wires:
  Upper Pendulum Encoder/1 -> Data Type Conversion/1
  Discrete Derivative/1 -> omega [rad/s]/1
  Data Type Conversion/1 -> Gain/1
  Gain/1 -> Discrete Derivative/1, phi [rad]/1

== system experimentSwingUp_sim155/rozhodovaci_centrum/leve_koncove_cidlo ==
  Inductive sensor LEFT : sldrtlib/Digital Input  SampleTime=Ts  MaxMissedTicks=1e6  ShowMissedTicks=off  YieldWhenWaiting=off  DrvName=Humusoft/MF624  DrvAddress=4294967295  DrvOptions=0  Channels=1  BitMode=1  DataType=1
  NOT : Logic  Operator=NOT  IconShape=distinctive  AllPortsSameDT=off  OutDataTypeStr=boolean
  NOK : Outport
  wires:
  Inductive sensor LEFT/1 -> NOT/1
  NOT/1 -> NOK/1

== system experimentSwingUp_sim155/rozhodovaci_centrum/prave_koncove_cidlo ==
  Inductive sensor RIGHT : sldrtlib/Digital Input  SampleTime=Ts  MaxMissedTicks=1e6  ShowMissedTicks=off  YieldWhenWaiting=off  DrvName=Humusoft/MF624  DrvAddress=4294967295  DrvOptions=0  Channels=2  BitMode=1  DataType=1
  NOT1 : Logic  Operator=NOT  IconShape=distinctive  AllPortsSameDT=off  OutDataTypeStr=boolean
  NOK : Outport
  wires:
  Inductive sensor RIGHT/1 -> NOT1/1
  NOT1/1 -> NOK/1

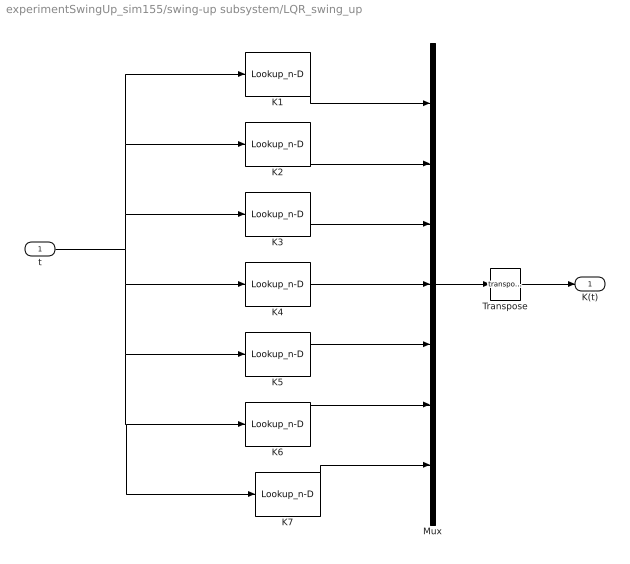
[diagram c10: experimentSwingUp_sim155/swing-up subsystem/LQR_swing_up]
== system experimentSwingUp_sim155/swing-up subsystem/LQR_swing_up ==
  t : Inport
  K1 : Lookup_n-D  NumberOfTableDimensions=1  BreakpointsForDimension1=t_FB  Table=K1  InternalRulePriority=Speed  RndMeth=Simplest
  K2 : Lookup_n-D  NumberOfTableDimensions=1  BreakpointsForDimension1=t_FB  Table=K2  InternalRulePriority=Speed  RndMeth=Simplest
  K3 : Lookup_n-D  NumberOfTableDimensions=1  BreakpointsForDimension1=t_FB  Table=K3  InternalRulePriority=Speed  RndMeth=Simplest
  K4 : Lookup_n-D  NumberOfTableDimensions=1  BreakpointsForDimension1=t_FB  Table=K4  InternalRulePriority=Speed  RndMeth=Simplest
  K5 : Lookup_n-D  NumberOfTableDimensions=1  BreakpointsForDimension1=t_FB  Table=K5  InternalRulePriority=Speed  RndMeth=Simplest
  K6 : Lookup_n-D  NumberOfTableDimensions=1  BreakpointsForDimension1=t_FB  Table=K6  InternalRulePriority=Speed  RndMeth=Simplest
  K7 : Lookup_n-D  NumberOfTableDimensions=1  BreakpointsForDimension1=t_FB  Table=Ki  InternalRulePriority=Speed  RndMeth=Simplest
  Mux : Mux  Inputs=7
  Transpose : Math  Operator=transpose
  K(t) : Outport  VectorParamsAs1DForOutWhenUnconnected=on
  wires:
  K5/1 -> Mux/5
  K1/1 -> Mux/1
  K2/1 -> Mux/2
  K6/1 -> Mux/6
  t/1 -> K7/1, K6/1, K5/1, K4/1, K3/1, K2/1, K1/1
  K4/1 -> Mux/4
  K3/1 -> Mux/3
  Mux/1 -> Transpose/1
  Transpose/1 -> K(t)/1
  K7/1 -> Mux/7

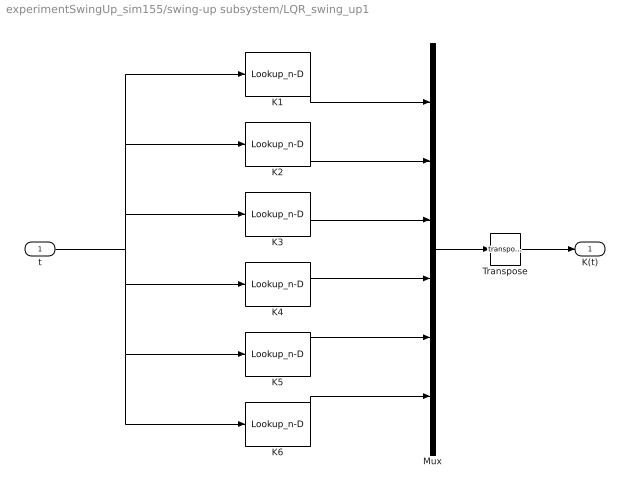
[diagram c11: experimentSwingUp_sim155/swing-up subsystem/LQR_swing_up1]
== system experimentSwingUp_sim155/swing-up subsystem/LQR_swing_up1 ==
  t : Inport
  K1 : Lookup_n-D  NumberOfTableDimensions=1  BreakpointsForDimension1=t_FB  Table=K1  InternalRulePriority=Speed  RndMeth=Simplest
  K2 : Lookup_n-D  NumberOfTableDimensions=1  BreakpointsForDimension1=t_FB  Table=K2  InternalRulePriority=Speed  RndMeth=Simplest
  K3 : Lookup_n-D  NumberOfTableDimensions=1  BreakpointsForDimension1=t_FB  Table=K3  InternalRulePriority=Speed  RndMeth=Simplest
  K4 : Lookup_n-D  NumberOfTableDimensions=1  BreakpointsForDimension1=t_FB  Table=K4  InternalRulePriority=Speed  RndMeth=Simplest
  K5 : Lookup_n-D  NumberOfTableDimensions=1  BreakpointsForDimension1=t_FB  Table=K5  InternalRulePriority=Speed  RndMeth=Simplest
  K6 : Lookup_n-D  NumberOfTableDimensions=1  BreakpointsForDimension1=t_FB  Table=K6  InternalRulePriority=Speed  RndMeth=Simplest
  Mux : Mux  Inputs=6
  Transpose : Math  Operator=transpose
  K(t) : Outport  VectorParamsAs1DForOutWhenUnconnected=on
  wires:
  K5/1 -> Mux/5
  K1/1 -> Mux/1
  K2/1 -> Mux/2
  K6/1 -> Mux/6
  t/1 -> K6/1, K5/1, K4/1, K3/1, K2/1, K1/1
  K4/1 -> Mux/4
  K3/1 -> Mux/3
  Mux/1 -> Transpose/1
  Transpose/1 -> K(t)/1

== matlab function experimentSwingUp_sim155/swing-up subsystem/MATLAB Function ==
function u = feedbackLinearization_pn155(y, v)
%feedbackLinearization: castecna feedback linearizace - ziskani vstupu pro nelinearni system

if y(4) >=  0 % pro kladne rychlosti b_0 = bp_0
    
    u = (407227096910748504076914119243960960953492563523831375978747126050092199441462516336971030531937534480482304000000*sin(2*y(3)) - 11500407088910324146229444568754977472486398737404017444437732424056822108965631195323726200028988324684156570173440*sin(2*y(2)) - 24184244866195054101831323117292646123759848193394465013263812327464634161494839357636883186990957753478963789824000*v - 61559052228213972062663301194102384707391699514339370480560408675933183962861907800345768722152915259906253127680000*y(4) + 1172314687962316426730830231269620537460387231131907996374896271565425291433805422561032232418857117704806989824000*v*cos(2*y(2)) - 41511426800280173708146189525378283481497712897434391027395221819581263959374364560343632062378953565798400000000*v*cos(2*y(3)) + 492045723340722615495028011226454017452946366853739292052179612616638111902587083211769291479153157578833218567541*y(5)^2*sin(y(2)) + 50295857773834799189479864038880676635514908862422130557322253979452276518744379794851283378667411165394501632000*y(6)^2*sin(y(3)) + 4886381360711363117555394466859569762199342131718374278066622500222385421803805633259156667162715121254400000000000*v*cos(2*y(2) - 2*y(3)) + 7263050669987173942265987748836687610041066651788929085738879757556545879587283107325219312762880000000000000000*cos(2*y(2) - y(3))*y(5) + 12949629628915619537830377839654122124111891749185519908491670983456792472947198031448048687158132736000000000000000*cos(2*y(2) - 2*y(3))*y(4) - 7263050669987173942265987748836687610041066651788929085738879757556545879587283107325219312762880000000000000000*cos(2*y(2) - y(3))*y(6) + 9598375883327782360522300495416211152969762948065962014481980256228086771971518560933848655035928202444800000000*sin(y(2) - 2*y(3))*y(5)^2 + 22282331604835469067702428897433847264384452559489323601535491529380520538303306109460532984911023308800000000000*y(5)*cos(y(2)) - 6178224845503107713832181816779954459693611170215349909809604911723664888652117385880781865730703360000000000000*y(5)*cos(y(3)) - 9017716265682905405409027352953892971060347895536436742159557775367226695516784382665165340536523980800000000000*y(6)*cos(y(2)) + 6178224845503107713832181816779954459693611170215349909809604911723664888652117385880781865730703360000000000000*y(6)*cos(y(3)) + 64496908227243814717814088608977115510649855854183576524253318118857625462989267473669950699504969770336256000000*y(6)^2*sin(2*y(2) - y(3)) - 4270195300250416688401631268211930494099518640040372875987811061856265168098600038736183951360000000000000000000*cos(y(2) - 2*y(3))*y(5) + 1728158897354997701608804393581124427815894932443086303985916132599091409916404886843173109760000000000000000000*cos(y(2) - 2*y(3))*y(6))/(15845632502852867518708790067200000000*(239006967539396035935973030594274634756909155463627229724502722981906396484375*cos(2*y(2) - 2*y(3)) - 1136174764783351394902810531656107874226455178782169636600620141135272382496583));
    
else % pro zaprone rychlosti b_0 = bn_0
    
    u = (407227096910748504076914119243960960953492563523831375978747126050092199441462516336971030531937534480482304000000*sin(2*y(3)) - 11500407088910324146229444568754977472486398737404017444437732424056822108965631195323726200028988324684156570173440*sin(2*y(2)) - 24184244866195054101831323117292646123759848193394465013263812327464634161494839357636883186990957753478963789824000*v - 33128070659239180531835972429230485216293237293111419185587461762520004623771589665550331654325031254863128821760000*y(4) + 1172314687962316426730830231269620537460387231131907996374896271565425291433805422561032232418857117704806989824000*v*cos(2*y(2)) - 41511426800280173708146189525378283481497712897434391027395221819581263959374364560343632062378953565798400000000*v*cos(2*y(3)) + 492045723340722615495028011226454017452946366853739292052179612616638111902587083211769291479153157578833218567541*y(5)^2*sin(y(2)) + 50295857773834799189479864038880676635514908862422130557322253979452276518744379794851283378667411165394501632000*y(6)^2*sin(y(3)) + 4886381360711363117555394466859569762199342131718374278066622500222385421803805633259156667162715121254400000000000*v*cos(2*y(2) - 2*y(3)) + 7263050669987173942265987748836687610041066651788929085738879757556545879587283107325219312762880000000000000000*cos(2*y(2) - y(3))*y(5) + 6968857216438344547586253988461834328832887435345326582521429467042623879001590705017855815295434752000000000000000*cos(2*y(2) - 2*y(3))*y(4) - 7263050669987173942265987748836687610041066651788929085738879757556545879587283107325219312762880000000000000000*cos(2*y(2) - y(3))*y(6) + 9598375883327782360522300495416211152969762948065962014481980256228086771971518560933848655035928202444800000000*sin(y(2) - 2*y(3))*y(5)^2 + 22282331604835469067702428897433847264384452559489323601535491529380520538303306109460532984911023308800000000000*y(5)*cos(y(2)) - 6178224845503107713832181816779954459693611170215349909809604911723664888652117385880781865730703360000000000000*y(5)*cos(y(3)) - 9017716265682905405409027352953892971060347895536436742159557775367226695516784382665165340536523980800000000000*y(6)*cos(y(2)) + 6178224845503107713832181816779954459693611170215349909809604911723664888652117385880781865730703360000000000000*y(6)*cos(y(3)) + 64496908227243814717814088608977115510649855854183576524253318118857625462989267473669950699504969770336256000000*y(6)^2*sin(2*y(2) - y(3)) - 4270195300250416688401631268211930494099518640040372875987811061856265168098600038736183951360000000000000000000*cos(y(2) - 2*y(3))*y(5) + 1728158897354997701608804393581124427815894932443086303985916132599091409916404886843173109760000000000000000000*cos(y(2) - 2*y(3))*y(6))/(15845632502852867518708790067200000000*(239006967539396035935973030594274634756909155463627229724502722981906396484375*cos(2*y(2) - 2*y(3)) - 1136174764783351394902810531656107874226455178782169636600620141135272382496583));
    
end

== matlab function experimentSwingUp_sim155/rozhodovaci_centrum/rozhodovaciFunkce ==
function [state, error] = rozhodovaciFunkce(last_state, leftSens, rightSens, stavySystemu, traj)

% inicializace: state == 0
error = 0; % bezchybovy chod
state = last_state; % novy stav

th0 = stavySystemu(1); % poloha voziku
th1 = stavySystemu(2); % natoceni prvniho ramene
th2 = stavySystemu(3); % natoceni druheho ramene
dth1 = stavySystemu(5); % uhlova rychlost prvniho ramene
dth2 = stavySystemu(6); % uhlova rychlost druheho ramene

switch (state)
    
    case 0 % swing-up
        NOKSwUp = zeros(2,1);
        NOKSwUp(1) = abs(traj(2) - th1) >= deg2rad(10);
        NOKSwUp(2) = abs(traj(3) - th2) >= deg2rad(10);
        
        if sum(NOKSwUp) ~= 0 % pokud alespon jedna nepripustna odchylka 
            state = 101; % chybovy stav
            error = 1;
        end
        
        % detekce zamotani kabelu enkoderu
        if (abs(th1) >= deg2rad(240))
            state = 102; % chybovy stav
            error = 1;
            % detekce inverzni polohy kyvadel
        elseif ((abs(th1) < deg2rad(5)) && (abs(th2) < deg2rad(5)) && (abs(dth1) < deg2rad(30)) && (abs(dth2) < deg2rad(30)))
            state = 1; % stabilizace
        end
        
        
        
    case 1 % stabilizace v inverzni poloze
        % detekce neuspesne stabilizace
        if ((abs(th1) >= deg2rad(30)) || (abs(th2) >= deg2rad(30)))
            state = 103; % chybovy stav
            error = 1;
        end
        
        
        
    otherwise % chybove stavy
        error = 1;
end

% detekce nebezpecne pozice (provest vzdy)
if (abs(th0) >= 0.5)
    state = 104; % chybovy stav
    error = 1;
end

% ochrana proti vyjeti voziku (provest vzdy)
if leftSens || rightSens
    state = 105; % chybovy stav
    error = 1;
end

end

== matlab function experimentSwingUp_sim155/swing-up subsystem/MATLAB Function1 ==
function on = feedbackOn(time)

on = 0;

if (time <= 0.9)  ||  (time >= 0.91)
    on = 1;
end
